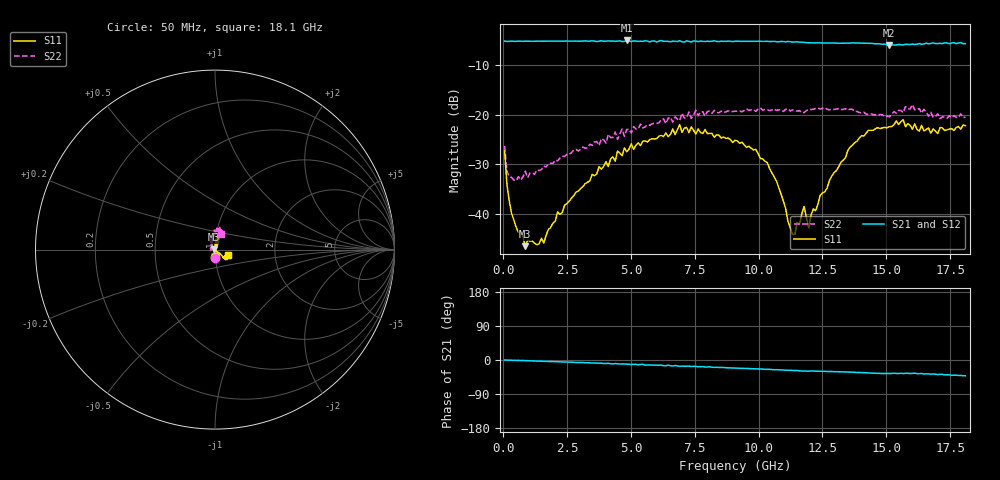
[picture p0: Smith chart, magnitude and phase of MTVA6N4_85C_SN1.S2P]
! Network Analyzer HP8720D.06.14 Serial No. US36140669
!  6 Jul 2005  07:30:40
! Frequency  S11  S21  S12  S22
# HZ  S  DB R 50
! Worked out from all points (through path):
!   201 points, 50 MHz to 18.1 GHz, reference 50 ohm
!   highest |S21| = -5.09 dB at 4.833 GHz (marker M1); lowest = -6.0 dB at 15.12 GHz (marker M2)
!   group delay of S21, straight-line fit = 6.44 ps
!   lowest |S11| = -46.5 dB at 862.2 MHz (marker M3), VSWR 1.01, Z = 49.5 + j0.123 ohm
!   |S11| at or under -10 dB: start of sweep to end of sweep
!   |S22| runs from -33.3 to -18.0 dB; largest |S21 - S12| = 0.017
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5e7  -27.34 -91.2  -5.21 -0.1  -5.24 0.2  -26.32 -91.9
1.4025e8  -34.03 -101.3  -5.29 -0.2  -5.26 -0.2  -31.35 -135.4
3.2075e8  -39.84 -125.0  -5.22 -0.5  -5.24 -0.5  -32.63 -164.8
8.6225e8  -46.47 164.9  -5.23 -1.7  -5.24 -1.7  -31.39 163.9
1.58425e9  -45.83 108.6  -5.23 -3.4  -5.22 -3.4  -30.34 137.8
2.12575e9  -39.59 77.6  -5.20 -4.7  -5.22 -4.7  -29.30 122.8
3.1185e9  -34.48 73.6  -5.19 -6.7  -5.23 -7.0  -26.54 119.9
4.47225e9  -27.34 64.1  -5.22 -10.1  -5.18 -9.6  -25.00 110.8
4.83325e9  -27.50 73.5  -5.09 -10.8  -5.15 -11.5  -23.00 97.2
6.09675e9  -24.33 70.8  -5.21 -13.8  -5.11 -14.0  -21.67 91.8
6.909e9  -22.01 76.5  -5.14 -16.8  -5.21 -15.9  -21.21 82.4
9.075e9  -25.16 82.7  -5.24 -21.2  -5.22 -21.2  -19.30 75.0
1.03385e10  -29.65 91.0  -5.26 -24.7  -5.28 -24.8  -19.01 70.0
1.133125e10  -44.13 38.6  -5.42 -27.4  -5.38 -27.6  -19.03 74.2
1.17825e10  -38.49 -70.9  -5.46 -29.0  -5.47 -29.4  -19.59 79.1
1.1963e10  -42.78 -84.5  -5.55 -29.6  -5.59 -29.5  -19.00 82.6
1.21435e10  -38.96 -51.8  -5.59 -29.0  -5.53 -29.1  -18.93 81.6
1.35875e10  -26.54 -40.1  -5.62 -31.9  -5.57 -32.0  -18.90 80.2
1.512175e10  -22.43 -38.5  -6.01 -35.7  -5.87 -35.6  -20.45 90.7
1.566325e10  -21.03 -37.9  -5.98 -35.7  -5.90 -34.7  -19.60 84.7
1.602425e10  -22.95 -41.4  -5.80 -35.4  -5.92 -36.6  -17.97 77.9
1.81e10  -22.22 -24.1  -5.73 -41.6  -5.84 -41.9  -20.50 69.8
